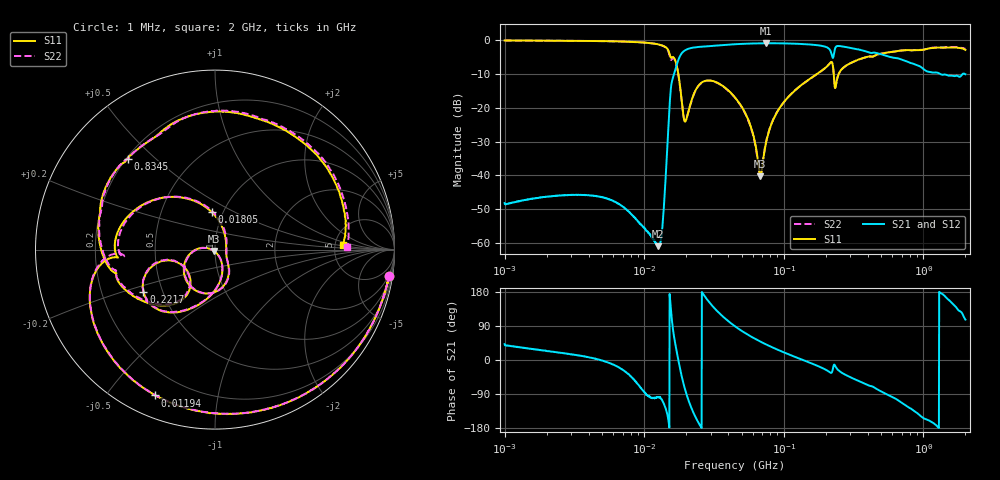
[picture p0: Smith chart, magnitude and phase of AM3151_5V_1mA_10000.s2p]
! Date/Time: Fri Jun 26 10:50:55 2020
! Network Analyzer:  Rev:
! Sweep from 1000000.0 to 2000000000.0, 1601 Points ! Power Supply: 0 V, 0 A
# HZ S DB R 50
!freq MagS11 AngS11 MagS21 AngS21 MagS12 AngS12 MagS22 AngS22
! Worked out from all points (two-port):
!   1601 points, 1 MHz to 2 GHz, reference 50 ohm
!   highest |S21| = -0.99 dB at 74.7 MHz (marker M1); lowest = -60.9 dB at 12.58 MHz (marker M2)
!   |S21| within 3 dB of the highest: 18.54 MHz to 219.2 MHz (200.7 MHz wide, 169 % of centre); 229.1 MHz to 474 MHz (244.9 MHz wide, 69.7 % of centre)
!   lowest |S11| = -40.3 dB at 67.93 MHz (marker M3), VSWR 1.02, Z = 49.4 - j0.726 ohm
!   |S11| at or under -10 dB: 17.55 MHz to 173.8 MHz (156.2 MHz wide, 163 % of centre); 227.8 MHz to 247.7 MHz (19.9 MHz wide, 8.37 % of centre)
!   |S22| runs from -40.4 to -0.2 dB; largest |S21 - S12| = 0.0076
!   S11 on the Smith chart (normalised r, x): 1 MHz: 2, -13; 11.94 MHz: 0.09, -0.67; 18.05 MHz: 0.88, +0.39; 221.7 MHz: 0.39, -0.24; 834.5 MHz: 0.20, +0.41; 2 GHz: 5.86, +0.57
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1000000  -0.17 -8.7  -48.15 41.9  -48.51 38.7  -0.17 -8.7
3555161  -0.29 -29.7  -45.77 10.7  -45.75 10.7  -0.29 -29.7
7113418  -0.48 -60.5  -49.34 -27.5  -49.31 -27.2  -0.49 -60.8
1.19388e7  -1.12 -112.3  -59.57 -99.5  -59.67 -99.6  -1.16 -113.0
1.257926e7  -1.31 -121.2  -60.88 -97.7  -60.77 -96.6  -1.33 -122.1
1.263916e7  -1.32 -122.2  -60.77 -97.8  -60.61 -97.7  -1.36 -123.0
1.363731e7  -1.72 -138.6  -53.07 -111.2  -53.01 -110.9  -1.77 -139.9
1.565164e7  -5.30 -175.4  -13.15 120.9  -13.15 120.9  -5.84 -175.4
1.804903e7  -13.51 95.3  -4.77 -22.1  -4.77 -22.1  -13.73 91.9
2.051914e7  -21.91 -35.5  -2.69 -100.7  -2.69 -100.7  -21.89 -35.7
2.528932e7  -12.88 -85.1  -2.03 -174.4  -2.03 -174.5  -12.95 -83.2
3.29969e7  -12.53 -132.1  -1.67 130.7  -1.67 130.7  -12.60 -130.8
4.493426e7  -17.08 -170.9  -1.27 88.5  -1.27 88.4  -17.17 -170.0
6.793144e7  -40.31 -130.4  -1.03 48.6  -1.02 48.5  -40.42 -123.7
7.470228e7  -30.24 -61.4  -0.99 41.1  -1.00 41.1  -30.02 -60.5
1.589914e8  -11.08 -99.5  -1.41 -9.4  -1.40 -9.5  -11.09 -99.8
2.217143e8  -6.67 -149.2  -4.74 -31.7  -4.74 -31.7  -6.69 -149.5
2.438128e8  -10.75 -121.9  -1.79 -25.8  -1.79 -25.7  -10.77 -123.0
5.652395e8  -3.65 171.1  -4.94 -93.2  -4.90 -93.2  -3.65 169.0
8.344696e8  -3.06 133.9  -6.93 -131.2  -6.89 -131.2  -3.04 131.3
1.354725e9  -2.29 75.4  -10.26 175.0  -10.20 174.5  -2.20 72.6
2e9  -2.96 1.9  -10.14 106.6  -10.29 105.9  -2.64 1.0
